|Texas Instruments Incorporated
|tmux8109, 100V 2 Channel 4:1 mux
[IBIS Ver]   4.1
[File name]   tmux8109.ibs
[Date]   08/12/21
[File Rev]   1.0
[Source]
| Texas Instruments Incorporated.
| ASC-INT-MPD
| 12500 TI Blvd
| Dallas, TX - 75243
[Notes]   Revision History:
| Rev 1.0: 08/12/21
| - Initial version of the model
| - Model generated from simulations in SPECTRE
| - C_comp although listed in numerical order of value are
|   obtained from varying PVT conditions. For PVT conditions for
|   each specific value refer the buffer description under
|   respective [Model]. IBIS model user is responsible for using
|   appropriate C_comp to simulate for Signal Integrity.
[Disclaimer]
| This model is designed as an aid for customers of Texas Instruments.
| TI and its licensors and suppliers make no warranties, either expressed
| or implied, with respect to this  model, including the warranties of
| merchantability or fitness for a particular purpose. The model is
| provided solely on an "as is" basis. The entire risk as to its quality
| and performance is with the customer.
| This model is subject to change without notice. Texas Instruments
| Incorporated is not responsible for updating this model.
[Copyright]
(C) Copyright 2021 Texas Instruments Incorporated.All rights reserved.
|  Component TMUX8109PW 15-pin - PW package
|  Part # TMUX8109PW
[Component]   TMUX8109PW
[Manufacturer]  TI
[Package]
|   typ   min   max
R_pkg   0.14389   NA   NA
L_pkg   1.96144nH   NA   NA
C_pkg   0.37623pF   NA   NA
[Pin]   signal_name   model_name
   1   A0   inbuf
   2   EN   inbuf
   3   VSS   power
   4   S1A   sterm
   5   S2A   sterm
   6   S3A   sterm
   7   S4A   sterm
   8   DA   dterm
   9   DB   dterm
   10   S4B   sterm
   11   S3B   sterm
   12   S1B   sterm
   13   VDD   power
   14   GND   gnd
   15   A1   inbuf
[Series Switch Groups]
On 1 /
On 2 /
On 3 /
On 4 /
Off 1 2 3 4 /
[Series Pin Mapping]  pin_2 model_name function_table_group
|   4   8   switch_dual_50   1
|  13   9   switch_dual_50   1
|   5   8   switch_dual_50   2
|  12   9   switch_dual_50   2
|   6   8   switch_dual_50   3
|  11   9   switch_dual_50   3
|   7   8   switch_dual_50   4
|  10   9   switch_dual_50   4
|   4   8   switch_dual_15   1
|  13   9   switch_dual_15   1
|   5   8   switch_dual_15   2
|  12   9   switch_dual_15   2
|   6   8   switch_dual_15   3
|  11   9   switch_dual_15   3
|   7   8   switch_dual_15   4
|  10   9   switch_dual_15   4
   4   8   switch_72   1
  13   9   switch_72   1
   5   8   switch_72   2
  12   9   switch_72   2
   6   8   switch_72   3
  11   9   switch_72   3
   7   8   switch_72   4
  10   9   switch_72   4
|   4   8   switch_100   1
|  13   9   switch_100   1
|   5   8   switch_100   2
|  12   9   switch_100   2
|   6   8   switch_100   3
|  11   9   switch_100   3
|   7   8   switch_100   4
|  10   9   switch_100   4
|   4   8   switch_dual_36   1
|  13   9   switch_dual_36   1
|   5   8   switch_dual_36   2
|  12   9   switch_dual_36   2
|   6   8   switch_dual_36   3
|  11   9   switch_dual_36   3
|   7   8   switch_dual_36   4
|  10   9   switch_dual_36   4
|  Component TMUX8109RUM 15-pin - RUM package
|  Part # TMUX8109RUM
[Component]   TMUX8109RUM
[Manufacturer]  TI
[Package]
|   typ   min   max
R_pkg   0.1   NA   NA
L_pkg   1.0nH   NA   NA
C_pkg   0.2pF   NA   NA
[Pin]   signal_name   model_name
   1   VSS   power
   2   S1A   sterm
   3   S2A   sterm
   4   S3A   sterm
   5   S4A   sterm
   6   DA   dterm
   7   DB   dterm
   8   S4B   sterm
   9   S3B   sterm
   10   S1B   sterm
   11   VDD   power
   12   GND   gnd
   13   A1   inbuf
   14   A0   inbuf
   15   EN   inbuf
[Series Switch Groups]
On 1 /
On 2 /
On 3 /
On 4 /
Off 1 2 3 4 /
[Series Pin Mapping]  pin_2 model_name function_table_group
|   2   6   switch_dual_50   1
|  11   7   switch_dual_50   1
|   3   6   switch_dual_50   2
|  10   7   switch_dual_50   2
|   4   6   switch_dual_50   3
|   9   7   switch_dual_50   3
|   5   6   switch_dual_50   4
|   8   7   switch_dual_50   4
|   2   6   switch_dual_15   1
|  11   7   switch_dual_15   1
|   3   6   switch_dual_15   2
|  10   7   switch_dual_15   2
|   4   6   switch_dual_15   3
|   9   7   switch_dual_15   3
|   5   6   switch_dual_15   4
|   8   7   switch_dual_15   4
|   2   6   switch_72   1
|  11   7   switch_72   1
|   3   6   switch_72   2
|  10   7   switch_72   2
|   4   6   switch_72   3
|   9   7   switch_72   3
|   5   6   switch_72   4
|   8   7   switch_72   4
|   2   6   switch_100   1
|  11   7   switch_100   1
|   3   6   switch_100   2
|  10   7   switch_100   2
|   4   6   switch_100   3
|   9   7   switch_100   3
|   5   6   switch_100   4
|   8   7   switch_100   4
|   2   6   switch_dual_36   1
|  11   7   switch_dual_36   1
|   3   6   switch_dual_36   2
|  10   7   switch_dual_36   2
|   4   6   switch_dual_36   3
|   9   7   switch_dual_36   3
|   5   6   switch_dual_36   4
|   8   7   switch_dual_36   4
[Model Selector] dterm
dterm_dual_50 Use for operation at +/-50V
dterm_dual_15 Use for operation at +/-15V
dterm_72 Use for operation at 72V
dterm_100 Use for operation at 100V
dterm_dual_36 Use for operation at +/-36V
[Model Selector] sterm
sterm_dual_50 Use for operation at +/-50V
sterm_dual_15 Use for operation at +/-15V
sterm_72 Use for operation at 72V
sterm_100 Use for operation at 100V
sterm_dual_36 Use for operation at +/-36V
[Model Selector] inbuf
inbuf_dual_50 Use for operation at +/-50V
inbuf_dual_15 Use for operation at +/-15V
inbuf_72 Use for operation at 72V
inbuf_100 Use for operation at 100V
inbuf_dual_36 Use for operation at +/-36V
| switch_dual_50
[Model]   switch_dual_50
Model_type   Series_switch
|   typ   min   max
C_comp   2.533030e-12   NA   NA
[Voltage Range]   50   NA   NA
[Power Clamp Reference]   50   NA   NA
[Temperature Range]   27   NA   NA
[On]
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[Off]
|   typ   min   max
[R Series]   10G   NA   NA
| switch_dual_15
[Model]   switch_dual_15
Model_type   Series_switch
|   typ   min   max
C_comp   4.014581e-12   NA   NA
[Voltage Range]   15   NA   NA
[Power Clamp Reference]   15   NA   NA
[Temperature Range]   27   NA   NA
[On]
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[Off]
|   typ   min   max
[R Series]   10G   NA   NA
| switch_72
[Model]   switch_72
Model_type   Series_switch
|   typ   min   max
C_comp   4.014581e-12   NA   NA
[Voltage Range]   72   NA   NA
[Power Clamp Reference]   72   NA   NA
[Temperature Range]   27   NA   NA
[On]
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[Off]
|   typ   min   max
[R Series]   10G   NA   NA
| switch_100
[Model]   switch_100
Model_type   Series_switch
|   typ   min   max
C_comp   4.014581e-12   NA   NA
[Voltage Range]   100   NA   NA
[Power Clamp Reference]   100   NA   NA
[Temperature Range]   27   NA   NA
[On]
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[Off]
|   typ   min   max
[R Series]   10G   NA   NA
| switch_dual_36
[Model]   switch_dual_36
Model_type   Series_switch
|   typ   min   max
C_comp   2.533030e-12   NA   NA
[Voltage Range]   36   NA   NA
[Power Clamp Reference]   36   NA   NA
[Temperature Range]   27   NA   NA
[On]
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[Off]
|   typ   min   max
[R Series]   10G   NA   NA
| Models and submodels in the file (20): dterm_dual_50 (Terminator), dterm_dual_15 (Terminator), dterm_72 (Terminator), dterm_100 (Terminator), dterm_dual_36 (Terminator), switch_dual_50 (Series_switch), switch_dual_15 (Series_switch), switch_72 (Series_switch), switch_100 (Series_switch), switch_dual_36 (Series_switch), sterm_dual_50 (Terminator), sterm_dual_15 (Terminator), sterm_72 (Terminator), sterm_100 (Terminator), sterm_dual_36 (Terminator), inbuf_dual_50 (Input), inbuf_dual_15 (Input), inbuf_72 (Input), inbuf_100 (Input), inbuf_dual_36 (Input)
